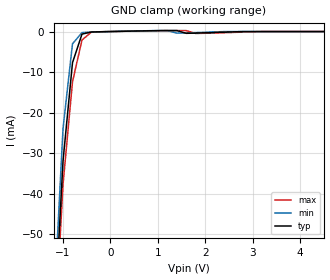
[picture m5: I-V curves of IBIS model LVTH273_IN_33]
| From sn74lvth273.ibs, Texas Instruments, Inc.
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|   Model LVTH273_IN_33
[Model]   LVTH273_IN_33
Model_type  Input
Polarity   Non-Inverting
Vinl = 0.8V
Vinh = 2.0V
| variable   typ   min   max
C_comp   4pf   NA   NA
[Temperature Range]   40   -25   100
| Ambient temperature   25   -40   85
[Voltage range]   3.3   3.0   3.6
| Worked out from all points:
|   GND clamp passes 1 mA (typ) near -0.61 V on its own axis
[GND Clamp]
|   Voltage   I(typ)   I(min)   I(max)
-5V       -1.683A    -1.921A    -1.491A
-1.2V     -75.83mA   -69.75mA   -80.79mA
-1V       -31.98mA   -23.97mA   -37.76mA
-800mV    -7.697mA   -3.024mA   -12.42mA
-600mV    -630.5uA   -250.4uA   -2.087mA
-400mV    -108.8uA   -118.5uA   -139.1uA
-200mV    -52.61uA   -58.26uA   -48.09uA
1.2V      242.7uA    248.4uA    231.3uA
1.4V      238.6uA    -397uA     245.2uA
1.6V      -438uA     -330.7uA   231.8uA
1.8V      -378.9uA   -252.5uA   -474.8uA
5V        -924.3pA   -35.94pA   -86.52pA
